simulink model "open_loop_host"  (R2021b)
settings: Solver=FixedStepDiscrete  StartTime=0.0  StopTime=Inf  RelTol=1e-3
undefined symbols (not defined in the file or in its folder): Serial
libraries: mcbhostblockslib x3

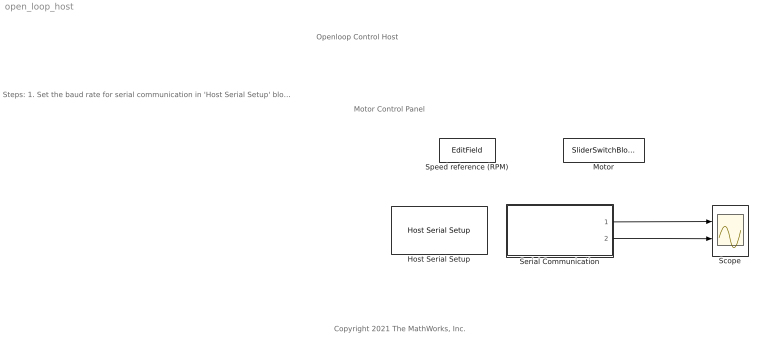
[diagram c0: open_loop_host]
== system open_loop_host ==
  note: Openloop Control Host
  note: Copyright 2021 The MathWorks, Inc.
  note: Steps: 1. Set the baud rate for serial communication in 'Host Serial Setup' block. 2. Select the serial port in ' Serial 1 ' tab of ' Host Serial Setup ' block. 3. Use ' Motor Start / Stop ' switch to control the motor. 4. Enter speed request in RPM using 'Speed Reference' edit box. Limit the reference speed to half of the rated speed. 5. Observe the ADC counts for phase current measurent in Scope.
  note: Motor Control Panel
  Host Serial Setup : mcbhostblockslib/Host Serial Setup  Priority=-99  comPortSer1='Please_select_a_port'  baudRateA=4000000  charLenA=8  stopBitA=1  parityA=none  timeoutA=2.0  ByteOrderA=LittleEndian  comPortSer2='Please_select_a_port'  baudRateB=115200  charLenB=8  stopBitB=1  parityB=none  timeoutB=1.0  ByteOrderB=LittleEndian  comPortSer3='Please_select_a_port'  baudRateC=115200  charLenC=8  stopBitC=1  parityC=none  timeoutC=1.0  ByteOrderC=LittleEndian  comPortSer4='Please_select_a_port'  baudRateD=115200  charLenD=8  stopBitD=1  parityD=none  timeoutD=1.0  ByteOrderD=LittleEndian
  Motor : SliderSwitchBlock  LabelPosition=Hide
  Scope : Scope  NumInputPorts=2
  Serial Communication : Subsystem
  Speed reference (RPM) : EditField  LabelPosition=Hide  ShowInitialText=on  Alignment=Center
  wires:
  Serial Communication/1(Ia (ADC)) -> Scope/1
  Serial Communication/2(Ib (ADC)) -> Scope/2

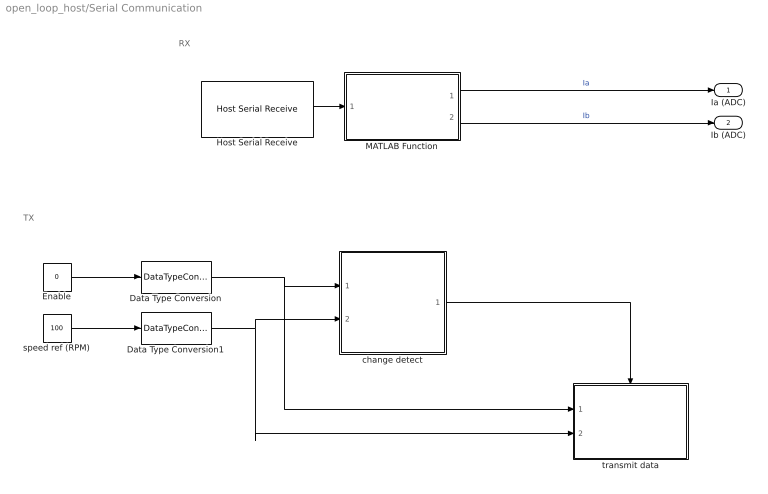
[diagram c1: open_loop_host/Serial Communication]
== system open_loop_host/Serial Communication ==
  note: TX
  note: RX
  Data Type Conversion : DataTypeConversion  OutDataTypeStr=single
  Data Type Conversion1 : DataTypeConversion  OutDataTypeStr=single
  Enable : Constant  Value=0  OutDataTypeStr=boolean  SampleTime=-1
  Host Serial Receive : mcbhostblockslib/Host Serial Receive  serialCon=Serial 1  dataHead='ss'  dataTail='ee'  dataType=uint16  dataDim=[200 2]  initValue=2000  errOption=Output custom value  errValue=4000  sampleTime=200 * 50e-6  outputStatus=off  blockingMode=on
  MATLAB Function : MATLAB Function  TreatAsAtomicUnit=on
  change detect : Subsystem
  speed ref (RPM) : Constant  Value=100  OutDataTypeStr=single  SampleTime=-1
  transmit data : Subsystem  TreatAsAtomicUnit=on
  Ia (ADC) : Outport
  Ib (ADC) : Outport  Port=2
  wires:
  Host Serial Receive/1 -> MATLAB Function/1(Input)
  MATLAB Function/1(Output1) -> Ia (ADC)/1  "Ia"
  MATLAB Function/2(Output2) -> Ib (ADC)/1  "Ib"
  Data Type Conversion1/1 -> transmit data/2(speed_ref_rpm), change detect/2(speed_ref_rpm)
  Data Type Conversion/1 -> transmit data/1(enable), change detect/1(enable)
  change detect/1(isChange) -> transmit data/Enable
  speed ref (RPM)/1 -> Data Type Conversion1/1
  Enable/1 -> Data Type Conversion/1

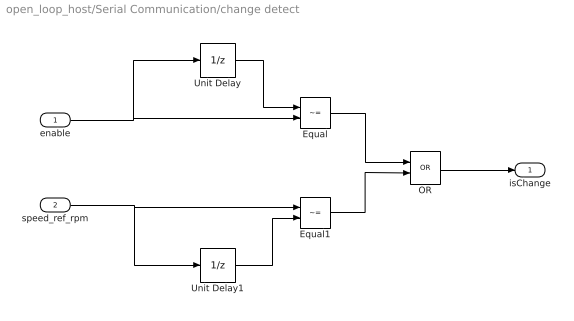
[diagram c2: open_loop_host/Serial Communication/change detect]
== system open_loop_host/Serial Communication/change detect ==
  enable : Inport
  speed_ref_rpm : Inport  Port=2
  Equal : RelationalOperator  Operator=~=  OutDataTypeStr=boolean  RndMeth=Simplest
  Equal1 : RelationalOperator  Operator=~=  OutDataTypeStr=boolean  RndMeth=Simplest
  OR : Logic  Operator=OR  AllPortsSameDT=off  OutDataTypeStr=boolean
  Unit Delay : UnitDelay  SampleTime=-1  HasFrameUpgradeWarning=on
  Unit Delay1 : UnitDelay  SampleTime=-1  HasFrameUpgradeWarning=on
  isChange : Outport
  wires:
  Unit Delay/1 -> Equal/1
  enable/1 -> Equal/2, Unit Delay/1
  speed_ref_rpm/1 -> Unit Delay1/1, Equal1/1
  Unit Delay1/1 -> Equal1/2
  OR/1 -> isChange/1
  Equal/1 -> OR/1
  Equal1/1 -> OR/2

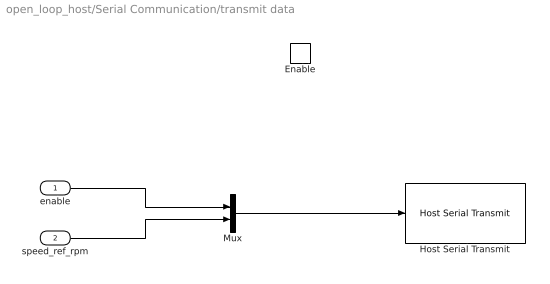
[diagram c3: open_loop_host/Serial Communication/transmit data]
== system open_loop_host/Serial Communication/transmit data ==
  enable : Inport
  speed_ref_rpm : Inport  Port=2
  Enable : EnablePort
  Host Serial Transmit : mcbhostblockslib/Host Serial Transmit  serialCon=Serial 1  header=''  tail=''  enableBlockingMode=off
  Mux : Mux  Inputs=2
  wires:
  enable/1 -> Mux/1
  speed_ref_rpm/1 -> Mux/2
  Mux/1 -> Host Serial Transmit/1

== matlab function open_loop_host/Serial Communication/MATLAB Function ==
function [ Output1, Output2] = unBuf(Input)

Output1 = Input(:, 1);
Output2 = Input(:, 2);
end
